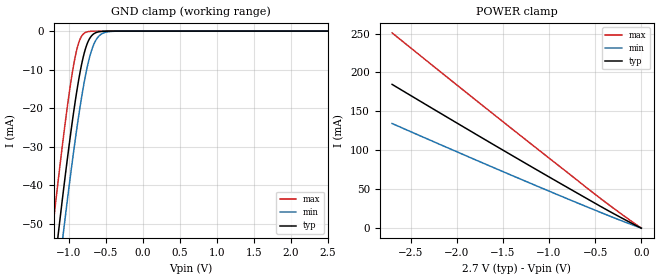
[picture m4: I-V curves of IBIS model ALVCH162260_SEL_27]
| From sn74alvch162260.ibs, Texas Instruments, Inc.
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[Model]   ALVCH162260_SEL_27
Model_type  Input
Vinl=0.8
Vinh=2.0
| variable   typ   min   max
C_comp   27.09pF   22.19pF   32.48pF
[Temperature Range]   40   100   -40
| Ambient temperature   25   85   -40
[Voltage range]   2.7   2.7   2.7
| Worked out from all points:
|   GND clamp passes 1 mA (typ) near -0.68 V on its own axis
|   POWER clamp passes 1 mA (typ) near -0.02 V on its own axis
[GND Clamp]
| ALVCH162260_SEL_27
|   Voltage   I(typ)   I(min)   I(max)
-2.5V     -300mA     -309.4mA   -288.3mA
-1.22V    -65.92mA   -76.78mA   -51.96mA
-1.15V    -54.2mA    -65.07mA   -40.19mA
-1.125V   -50.1mA    -60.96mA   -36.1mA
-1.07V    -41.27mA   -52.08mA   -27.39mA
-980mV    -27.63mA   -38.14mA   -14.46mA
-910mV    -18.08mA   -28.05mA   -6.523mA
-845mV    -10.58mA   -19.54mA   -2.069mA
-780mV    -5.041mA   -12.24mA   -440.8uA
-655mV    -630uA     -3.209mA   -15.41uA
-485mV    -21.18uA   -229.3uA   -148.8nA
2.5V      1.112nA    1.808uA    4.19pA
[POWER Clamp]
| ALVCH162260_SEL_27
|   Voltage   I(typ)   I(min)   I(max)
-2.7V     184.7mA    134.4mA    250.8mA
-1.58V    105.8mA    76.76mA    144.4mA
-565mV    36.32mA    26.23mA    49.42mA
-35.59fV  380pA      586.8pA    93.4pA
